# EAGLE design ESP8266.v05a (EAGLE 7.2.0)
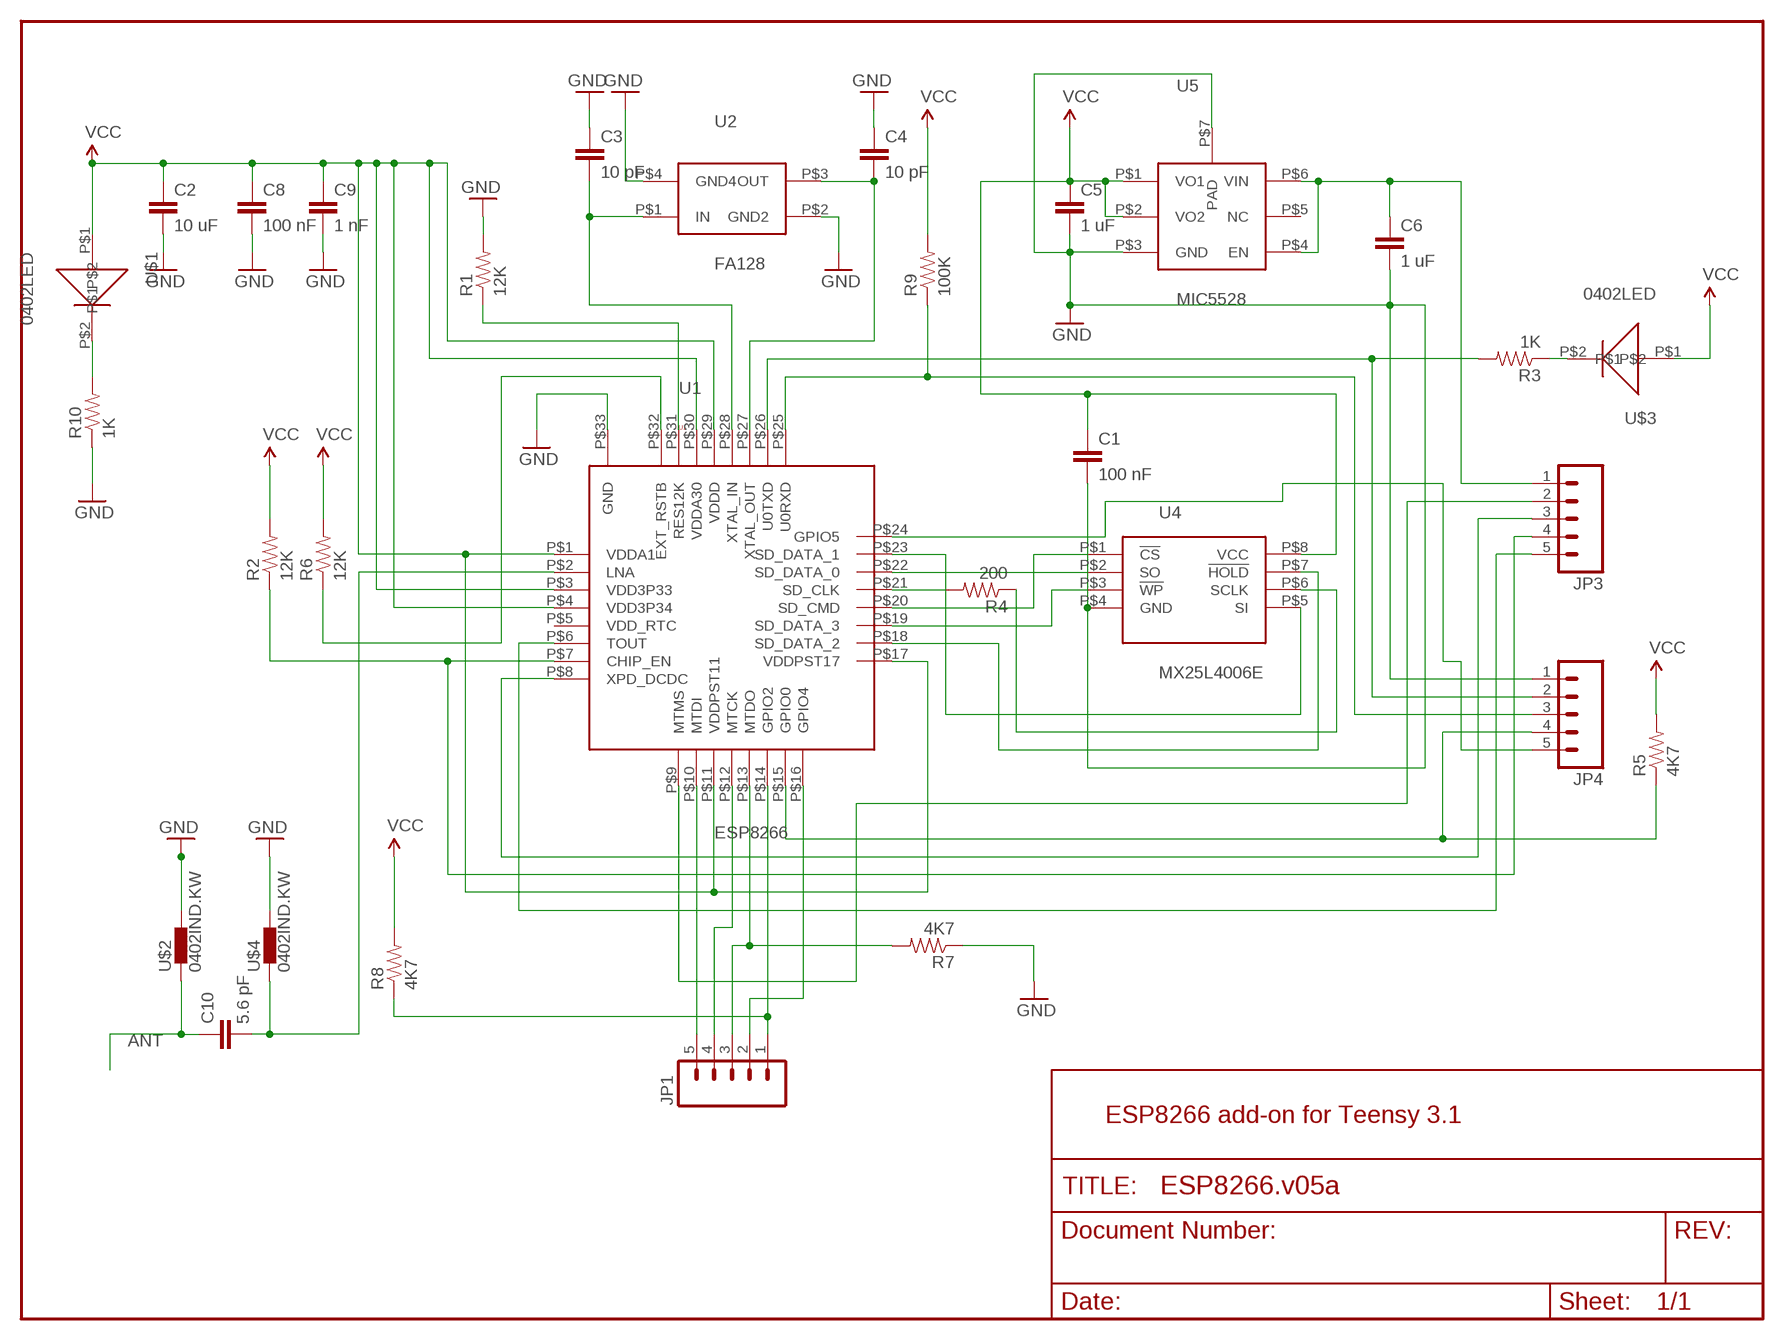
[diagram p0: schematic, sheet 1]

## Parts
C1  100 nF  0402CAP.KW  [0402-CAP]
C2  10 uF  0402CAP.KW  [0402-CAP]
C3  10 pF  0402CAP.KW  [0402-CAP]
C4  10 pF  0402CAP.KW  [0402-CAP]
C5  1 uF  0402CAP.KW  [0402-CAP]
C6  1 uF  0402CAP.KW  [0402-CAP]
C8  100 nF  0402CAP.KW  [0402-CAP]
C9  1 nF  0402CAP.KW  [0402-CAP]
C10  5.6 pF  0402CAP.KW  [0402-CAP]
JP1  M05NO_SILK  [1X05_NO_SILK]
JP3  M05NO_SILK  [1X05_NO_SILK]
JP4  M05NO_SILK  [1X05_NO_SILK]
R1  12K  0402RES.KW  [0402-RES]
R2  12K  0402RES.KW  [0402-RES]
R3  1K  0402RES.KW  [0402-RES]
R4  200  0402RES.KW  [0402-RES]
R5  4K7  0402RES.KW  [0402-RES]
R6  12K  0402RES.KW  [0402-RES]
R7  4K7  0402RES.KW  [0402-RES]
R8  4K7  0402RES.KW  [0402-RES]
R9  100K  0402RES.KW  [0402-RES]
R10  1K  0402RES.KW  [0402-RES]
U1  ESP8266  [ESP8266]
U2  FA128  [FA128]
U4  MX25L4006E  [USON-8]
U5  MIC5528  [MIC5528]
U$1  0402LED  [0402LED]
U$2  0402IND.KW  [0402]
U$3  0402LED  [0402LED]
U$4  0402IND.KW  [0402]

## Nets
ANT: C10.1 U$2.1
GND: C1.2 C2.2 C3.1 C4.1 C5.2 C6.2 C8.2 C9.2 JP4.1 R1.2 R7.1 R10.1 U1.P$33(GND) U2.P$2(GND2) U2.P$4(GND4) U4.P$4(GND) U5.P$3(GND) U5.P$7(PAD) U$2.2 U$4.2
N$1: C3.2 U1.P$28(XTAL_IN) U2.P$1(IN)
N$2: C4.2 U1.P$27(XTAL_OUT) U2.P$3(OUT)
N$3: C10.2 U1.P$2(LNA) U$4.1
N$4: JP3.3 U1.P$8(XPD_DCDC)
N$5: JP1.1 R8.1 U1.P$14(GPIO2)
N$6: JP4.4 R5.1 U1.P$15(GPIO0)
N$7: JP4.5 U1.P$24(GPIO5)
N$8: C6.1 JP3.1 U5.P$4(EN) U5.P$6(VIN)
N$9: JP4.2 R3.2 U1.P$26(U0TXD)
N$10: U1.P$23(SD_DATA_1) U4.P$5(SI)
N$11: JP4.3 R9.1 U1.P$25(U0RXD)
N$12: R10.2 U$1.P$2
N$13: R1.1 U1.P$31(RES12K)
N$14: R4.2 U1.P$21(SD_CLK)
N$15: R4.1 U4.P$6(SCLK)
N$16: U1.P$20(SD_CMD) U4.P$1(!CS)
N$17: U1.P$18(SD_DATA_2) U4.P$7(!HOLD)
N$18: JP3.2 U1.P$9(MTMS)
N$19: U1.P$19(SD_DATA_3) U4.P$3(!WP)
N$20: JP1.5 U1.P$10(MTDI)
N$21: U1.P$22(SD_DATA_0) U4.P$2(SO)
N$22: JP1.4 U1.P$12(MTCK)
N$23: JP1.3 R7.2 U1.P$13(MTDO)
N$24: JP1.2 U1.P$16(GPIO4)
N$25: JP3.4 R2.1 U1.P$7(CHIP_EN)
N$26: R3.1 U$3.P$2
N$28: R6.1 U1.P$32(EXT_RSTB)
N$29: JP3.5 U1.P$6(TOUT)
VCC: C1.1 C2.1 C5.1 C8.1 C9.1 R2.2 R5.2 R6.2 R8.2 R9.2 U1.P$1(VDDA1) U1.P$3(VDD3P33) U1.P$4(VDD3P34) U1.P$11(VDDPST11) U1.P$17(VDDPST17) U1.P$29(VDDD) U1.P$30(VDDA30) U4.P$8(VCC) U5.P$1(VO1) U5.P$2(VO2) U$1.P$1 U$3.P$1
Unconnected: U1.P$5(VDD_RTC) U5.P$5(NC)

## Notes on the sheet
- ESP8266 add-on for Teensy 3.1

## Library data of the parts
C1-C6 C8-C10 = SparkFun-Capacitors:0402CAP.KW
JP1 JP3 JP4 = SparkFun-Connectors:M05: Header 5 Standard 5-pin 0.1" header. Use with straight break away headers (SKU : PRT-00116), right angle break away headers (PRT-00553), swiss pins (PRT-00743), machine pins (PRT-00117), and female headers (PRT-00115). Molex polarized connector foot print use with SKU : PRT-08230 with associated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
R1-R10 = SparkFun-Resistors:0402RES.KW
U1 = Kris:ESP8266: QFN-32 package for espressif's ESP8266 WiFi microprocessor
U2 = Kris:FA128: FA-128 Espon crystal
U4 = Kris:MX25L4006E: uson-8 package for Macronix MX25L4006E 4 Mbit SPI Fash
U5 = Kris:MIC5528: MIC5528 500 mA 3.3V LDO voltage regulator by Micrel
U$1 U$3 = Kris:0402LED: 0402led
U$2 U$4 = inductors:0402IND.KW

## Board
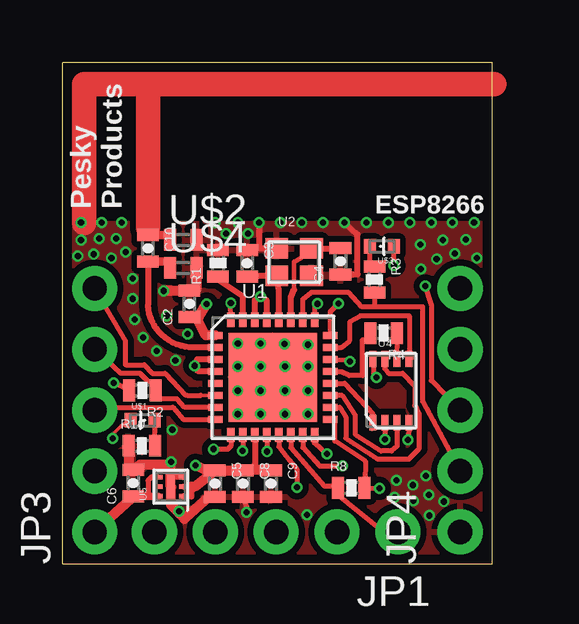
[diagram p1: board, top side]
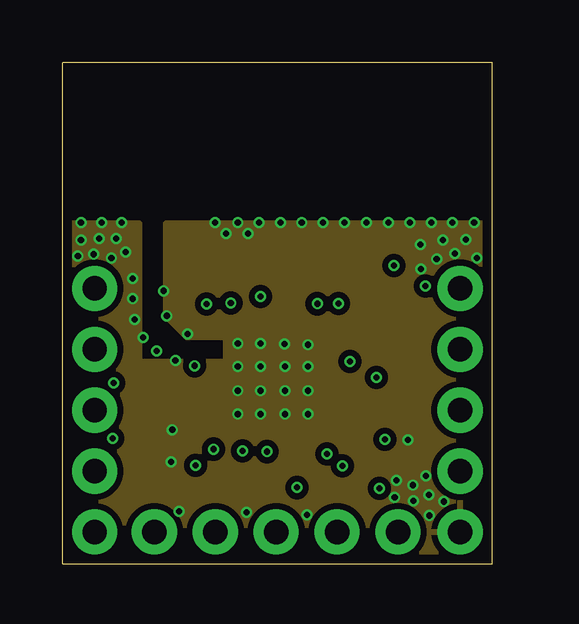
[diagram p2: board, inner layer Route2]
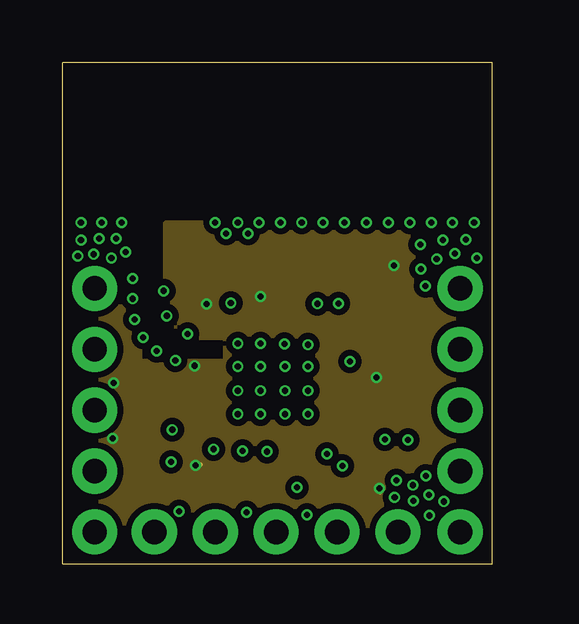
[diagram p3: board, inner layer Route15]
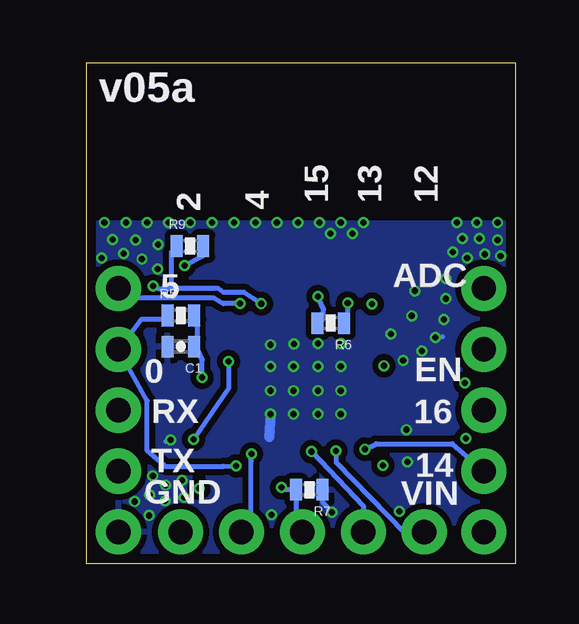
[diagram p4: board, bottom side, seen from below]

Size 17.91 x 20.9 mm. Coordinates in mm from the lower left corner, seen from the top.
Outline: 0,0 17.91,0 17.91,20.9 0,20.9 0,0
Copper layers (1*2*15*16): Top 0.035559375mm / dielectric 0.17018125mm / Route2 0.01778125mm / dielectric 47mil / Route15 0.01778125mm / dielectric 0.17018125mm / Bottom 0.035559375mm
Design rules "OSHPark-4layer *": minimum track width 5mil, minimum drill 10mil, track to track 5mil, track to pad 5mil, pad to pad 5mil, via to via 5mil, smd to smd 5mil, copper to edge 15mil, drill to drill 6mil, minimum pad ring 4mil, minimum via ring 4mil, stop-mask expansion 4mil, vias tented up to drill 20mil, thermal gap 10mil

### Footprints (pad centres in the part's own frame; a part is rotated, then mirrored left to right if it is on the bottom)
0402-CAP = smd 0.5 x 0.9: 1 -0.55,0; 2 0.55,0
1X05_NO_SILK = drill 1.016 pad 1.88: 1 0,0; 2 2.54,0; 3 5.08,0; 4 7.62,0; 5 10.16,0
0402-RES = smd 0.5 x 0.9: 1 -0.55,0; 2 0.55,0
ESP8266 = smd 0.6 x 0.3: P$1 -2.4,1.75; P$2 -2.4,1.25; P$3 -2.4,0.75; P$4 -2.4,0.25; P$5 -2.4,-0.25; P$6 -2.4,-0.75; P$7 -2.4,-1.25; P$8 -2.4,-1.75; P$17 2.4,-1.75; P$18 2.4,-1.25; P$19 2.4,-0.75; P$20 2.4,-0.25; P$21 2.4,0.25; P$22 2.4,0.75; P$23 2.4,1.25; P$24 2.4,1.75 | smd 0.3 x 0.6: P$9 -1.75,-2.4; P$10 -1.25,-2.4; P$11 -0.75,-2.4; P$12 -0.25,-2.4; P$13 0.25,-2.4; P$14 0.75,-2.4; P$15 1.25,-2.4; P$16 1.75,-2.4; P$25 1.75,2.4; P$26 1.25,2.4; P$27 0.75,2.4; P$28 0.25,2.4; P$29 -0.25,2.4; P$30 -0.75,2.4; P$31 -1.25,2.4; P$32 -1.75,2.4 | smd 3.7 x 3.7: P$33 0,0
FA128 = smd 0.95 x 0.85: P$1 -0.725,-0.575; P$2 0.725,-0.575; P$3 0.725,0.575; P$4 -0.725,0.575
USON-8 = smd 0.3 x 0.65: P$1 -0.75,-1.325; P$2 -0.25,-1.325; P$3 0.25,-1.325; P$4 0.75,-1.325; P$5 0.75,1.325; P$6 0.25,1.325; P$7 -0.25,1.325; P$8 -0.75,1.325
MIC5528 = smd 0.18 x 0.35: P$1 -0.4,-0.525; P$2 0,-0.525; P$3 0.4,-0.525; P$4 0.4,0.525; P$5 0,0.525; P$6 -0.4,0.525 | smd 0.94 x 0.3: P$7 0,0
0402LED = smd 0.5 x 0.6: P$1 -0.5,0; P$2 0.5,0
0402 = smd 0.5 x 0.9: 1 -0.55,0; 2 0.55,0

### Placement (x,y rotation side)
C1  13.97,9.07 180 bottom
C2  5.28,10.85 90 top
C3  7.7,12.55 270 top
C4  11.58,12.62 90 top
C5  6.35,3.35 270 top
C6  2.95,3.38 90 top
C8  7.52,3.35 270 top
C9  8.69,3.35 270 top
C10  3.56,13.16 270 top
JP1  13.98,1.33 180 top
JP3  1.33,1.33 90 top
JP4  16.57,1.33 90 top
R1  6.48,12.55 90 top
R2  3.33,7.24 180 top
R3  13,11.86 270 top
R4  13.39,9.63 180 top
R5  13.97,10.36 0 bottom
R6  7.72,10.05 180 bottom
R7  8.61,3.1 180 bottom
R8  12.04,3.17 0 top
R9  13.59,13.26 0 bottom
R10  3.3,4.93 0 top
U1  8.76,7.79 0 top
U2  9.65,12.59 0 top
U4  13.69,7.23 0 top
U5  4.51,3.23 90 top
U$1  3.34,5.99 0 top
U$2  5.03,13.51 0 top
U$3  13.31,13.25 180 top
U$4  5.03,12.34 0 top

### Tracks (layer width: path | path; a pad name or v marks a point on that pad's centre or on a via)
ANT
  Top 0.254: C10.1 3.58,14.01 3.56,14.04
  Top 0.356: C10.1 4.43,13.71 U$2.1
  Top 0.813: 3.56,14.04 3.56,14.31 | 18,20 18.01,20.04
  Top 1.016: 3.56,14.04 3.56,20 18,20
GND  (via drill 0.25)
  Top 0.203: 8.45,7.12 8.45,7.19 U1.P$33 | U4.P$4 14.41,5.04 v14.4,5.18 | v7.67,2.16 7.67,2.4 C8.2
  Top 0.254: U2.P$4 8.19,13.16 | 8.19,13.16 7.82,13.16 | v8.19,14.24 8.19,13.16 | 4.98,11.4 C2.2 5.58,11.46 | C4.1 12.1,12.07 12.29,12.09 12.29,13.74 v11.75,14.24 | v0.76,14.24 0.85,14.24 0.9,14.22 | U5.P$3 4.62,3.63 4.51,3.73
  Top 0.406: v8.26,8.24 v9.27,8.24 | v8.26,7.23 v9.27,7.23 | v8.26,8.24 8.26,7.29 | 8.26,7.29 v8.26,7.23 | v8.26,7.23 v7.3,7.23 v7.3,6.25 | v8.26,6.25 v8.26,7.23 | v9.27,6.25 v9.27,7.23 | v10.22,6.25 v10.22,7.23 v9.27,7.23 | v9.27,8.24 v9.25,9.17 v10.22,9.14 v10.22,8.24 | v8.26,8.24 v8.26,9.2 v7.3,9.2 v7.3,8.24 | v9.27,8.24 9.27,7.95 | 9.27,7.95 8.45,7.12 9.14,7.12 v9.27,7.23 | v9.27,7.23 9.27,7.95 | 9.27,7.95 8.45,7.95 8.32,8.08 8.32,7.12 8.26,7.29 | 4.29,11.41 4.98,11.4 | U$4.2 5.58,11.46 | R10.1 2.75,4.15 C6.2 3.21,4.14 4.5,4.14 4.51,4.18 4.51,3.73 U5.P$7 4.52,3.21 4.52,2.44 5.08,1.88 5.11,1.93 6.08,2.8 C5.2
  Top 0.813: 0.9,14.22 0.86,14.17
  Top 1.016: 3.43,20 0.9,20 0.9,14.22
  Bottom 0.203: 3.06,9.47 v3.35,9.45 | v14.4,5.18 14.61,5.11 | R7.1 8.06,2.57 v7.67,2.16
  Bottom 0.406: v10.22,6.25 10.29,5.28
  other vias: 9.97,14.24 15.38,14.24 13.58,14.24 17.16,14.24 6.35,14.24 2.46,14.24 2.63,13 2.92,11.06 1.63,14.24 7.3,14.24 9.08,14.24 10.86,14.24 14.48,14.24 16.26,14.24 12.66,14.24 4.22,11.39 4.34,10.35 4.7,8.49 15.85,13.5 16.81,13.53 15.29,2.02 4.52,4.25 3,10.2 3.91,8.88 2.92,11.9 2.24,13.58 2.03,12.76 1.52,13.58 0.76,13.5 0.64,12.84 15.6,12.71 16.36,12.94 17.27,12.76 10.19,2.04 4.57,5.6 1.3,12.92 5.21,9.59 6.82,13.78 7.73,13.78 15.9,2.6 15.14,3.67 13.84,2.78 13.92,3.49 14.63,2.63 14.61,3.29 15.27,2.88 14.91,13.32 14.94,12.31 4.85,2.2
  pour Top (isolate 0.254): 0,14.24 0,-0.03 17.91,-0.03 17.91,14.24
  pour Bottom (isolate 0.254): 0,14.24 -0.1,0 17.81,0 17.91,14.24
  pour Route2 (isolate 0.254): 0,14.24 3.2,14.24 3.2,8.46 6.78,8.46 6.78,9.42 5.18,9.42 4.29,10.31 4.29,14.24 17.91,14.24 17.91,0.03 0,0.03
N$1
  Top 0.254: U1.P$28 9.01,11.42 U2.P$1 C3.2
N$2
  Top 0.152: 9.95,12.78 U2.P$3
  Top 0.191: 9.65,11.44 9.65,12.6
  Top 0.203: 9.65,12.6 9.95,12.78 | 11.54,13.16 C4.2
  Top 0.254: U1.P$27 9.51,11.11 9.65,11.44 | U2.P$3 11.54,13.16
N$3
  Top 0.254: U1.P$2 5.26,9.04 arc-80 3.56,10.79 C10.2
  Top 0.356: C10.2 4.48,12.61 U$4.1
N$4
  Top 0.152: 6.18,6.03 U1.P$8
  Top 0.203: JP3.3 1.46,6.53 1.89,6.54 2.21,6.53 4.6,6.53 5.03,6.03 6.18,6.03
N$5
  Top 0.203: U1.P$14 9.51,4.85 10.9,3.25 11.19,3.25 R8.1 11.46,2.91 13.31,1.4 13.79,1.4 JP1.1
N$6  (via drill 0.25)
  Top 0.203: U1.P$15 10.01,4.86 10.72,4.09 v11.67,4.09
  Bottom 0.203: v11.67,4.09 12.19,4.08 14.66,4.08 14.66,4.09 15.37,4.72 15.37,6.81 JP4.4 15.63,10.19 14.68,10.19
  Bottom 0.254: 14.68,10.19 14.52,10.19 R5.1
N$7  (via drill 0.25)
  Top 0.203: U1.P$24 11.16,10.53 v11.49,10.86
  Bottom 0.203: v11.49,10.86 12.21,10.86 12.59,11.1 16.05,11.1 JP4.5
N$8
  Top 0.203: C6.1 | U5.P$4 3.7,3.63 3.56,3.48 3.56,2.9 3.48,2.83
  Top 0.305: U5.P$6 3.48,2.83 C6.1
  Top 0.406: JP3.1 2.86,2.72 C6.1
N$9
  Top 0.203: U1.P$26 10.01,11.04 10.35,11.32 11.94,11.32 12.48,10.72 13.06,10.72 | JP4.2 15.01,6.77 15.01,10.72 13.06,10.72 | R3.2 13.01,10.78 13.06,10.72
N$10
  Top 0.203: U1.P$23 11.63,9.04 11.95,9.3 11.96,9.35 11.96,10.08 12.41,10.35 14.45,10.35 14.45,8.59 U4.P$5 14.59,8.64 14.62,8.64
N$11  (via drill 0.25)
  Top 0.203: U1.P$25 10.51,10.78 v10.62,10.85 | JP4.3 15.37,7.64 15.37,10.82 v15.13,11.6
  Bottom 0.203: v10.62,10.85 11.33,11.33 12.19,11.33 12.39,11.48 14.36,11.48 | 14.32,12.95 R9.1 14.36,13.01 14.36,11.77 14.36,11.67 14.36,11.48 | v15.13,11.6 14.88,11.48 14.36,11.48
N$12
  Top 0.203: U$1.P$2 3.81,4.91 R10.2
N$13
  Top 0.254: U1.P$31 7.51,11.15 6.48,11.85 R1.1
N$14
  Top 0.152: 12.51,9.36 12.64,9.43 R4.2
  Top 0.203: 12.51,9.36 12.51,7.86 11.94,7.86 11.62,8.01 11.17,8.01 U1.P$21
N$15
  Top 0.152: 13.95,9.39 14.08,9.48 R4.1
  Top 0.203: U4.P$6 13.95,9.39
N$16
  Top 0.203: U1.P$20 11.76,7.54 12.93,6.25 12.93,5.78 12.9,5.65 12.9,5.92
  Top 0.254: 12.9,5.92 U4.P$1
N$17
  Top 0.203: U4.P$7 13.43,8.15 13.59,7.95 14.17,7.95 14.68,7.4 14.68,6.6 14.86,6.24 14.86,4.8 14.44,4.38 13.13,4.38 11.81,5.25 11.81,6.13 11.56,6.54 U1.P$18
N$18  (via drill 0.25)
  Top 0.203: U1.P$9 7.01,4.92 6.88,4.79 v6.29,4.79
  Bottom 0.203: v6.29,4.79 5.82,5.02 2.64,5.02 JP3.2
N$19
  Top 0.203: U4.P$3 13.94,4.91 13.72,4.71 13.27,4.71 12.19,5.41 12.19,6.21 11.66,7.02 11.16,7.02
  Top 0.254: 11.16,7.02 U1.P$19
N$20  (via drill 0.25)
  Top 0.203: U1.P$10 7.51,4.91 v7.51,4.71
  Bottom 0.203: v7.51,4.71 7.49,4.23 4.65,1.31 JP1.5
N$21  (via drill 0.25)
  Top 0.152: 13.44,5.96 13.51,5.95 U4.P$2
  Top 0.203: U1.P$22 11.89,8.51 v11.98,8.45 | 13.44,5.96 v13.44,5.19
  Bottom 0.203: v11.98,8.45 11.98,7.33 v13.44,5.19
N$22  (via drill 0.25)
  Top 0.203: U1.P$12 8.51,4.81 v8.52,4.69
  Bottom 0.203: v8.52,4.69 6.35,2.4 JP1.4
N$23  (via drill 0.25)
  Top 0.203: U1.P$13 9.01,4.89 9.46,4.33 9.77,3.95 v9.77,3.19
  Bottom 0.203: v9.77,3.19 9.77,3.1 R7.2 9.16,1.57 JP1.3
N$24  (via drill 0.25)
  Top 0.203: 10.51,5.06 v11.02,4.58
  Top 0.254: U1.P$16 10.51,5.06
  Bottom 0.203: v11.02,4.58 11.04,4.28 11.04,1.74 11.28,1.47 11.33,1.45 JP1.2
N$25
  Top 0.152: R2.1 3.99,7.45 3.72,7.45
  Top 0.203: U1.P$7 5.08,6.54 4.76,6.88 4.11,6.88 R2.1 | 3.72,7.45 3.23,7.95 2.41,7.95 JP3.4
N$26
  Top 0.203: R3.1 12.81,12.56 U$3.P$2
N$28  (via drill 0.25)
  Top 0.203: U1.P$32 v7.01,10.88
  Bottom 0.203: R6.1 7.02,10.13 v7.01,10.88
N$29
  Top 0.152: U1.P$6 5.77,7.04 | 5.13,7.04 5.18,7.04
  Top 0.203: JP3.5 2.62,9.31 2.62,8.31 3.4,8.31 3.73,7.95 4.27,7.95 5.13,7.04 | 5.18,7.04 5.77,7.04
VCC  (via drill 0.25)
  Top 0.152: R2.2 2.7,7.28 2.7,7.3 | U$1.P$1 2.41,5.74 2.14,5.46 2.14,5.29 v2.08,5.23
  Top 0.203: U1.P$17 11.19,6.01 11.35,6.01 11.35,5.13 12.62,4.29 12.61,3.38 R8.2 v13.21,3.15 | 2.7,7.3 v2.12,7.56 | U4.P$8 12.97,7.86 v13.08,7.77 | C5.1 6.04,3.86 | U$3.P$1 13.8,13 v13.82,12.45
  Top 0.254: U1.P$29 8.51,10.98 v8.26,11.15 8.01,11 U1.P$30 | 6.35,9.54 U1.P$1 | U1.P$3 5.61,8.54 v5.5,8.27 5.66,8.04 U1.P$4 | U1.P$11 8.01,4.18 8.01,3.94 | 8.6,3.94 C9.1 | C8.1 7.5,3.93 | U5.P$2 5.36,3.23 5.36,2.82 5.03,2.82 U5.P$1
  Top 0.406: 8.6,3.94 8.01,3.94 7.5,3.93 | 6.04,3.86 v5.54,4.12 | C8.1 C5.1 5.5,3.23 5.36,3.23 | U1.P$1 5.96,9.54 5.59,10.29 C2.1 5.67,10.3 v5.99,10.85
  Route15 0.203: v2.08,5.23 2.06,5.18 | v5.54,4.12 5.74,4.14 | v13.21,3.15 13.18,3.1 13.23,3
  Route15 0.254: 5.99,10.79 v5.99,10.85 6.02,10.82
  Bottom 0.203: v13.08,7.77 13.08,8.49 13.42,9.21 C1.1 13.27,9.4 13.27,10.21 R5.2 | R6.2 8.17,10.08 8.01,10.24 8.01,10.63 v8.26,11.15 | R9.2 13.04,12.84 v13.82,12.45
  Bottom 0.254: 13.37,10.41 13.42,10.39 R5.2
  pour Route15 (isolate 0.254): 0,14.24 3.2,14.24 3.2,8.46 6.78,8.46 6.78,9.42 5.18,9.42 4.29,10.31 4.29,14.24 17.91,14.24 17.83,0.03 -0.08,0.03

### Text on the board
tPlace: Pesky / Products | ESP8266
bPlace: v05a | 12 | 13 | 15 | 4 | 2 | ADC | 5 | EN | 0 | 16 | RX | 14 | TX | GND | VIN
tValues: DNP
